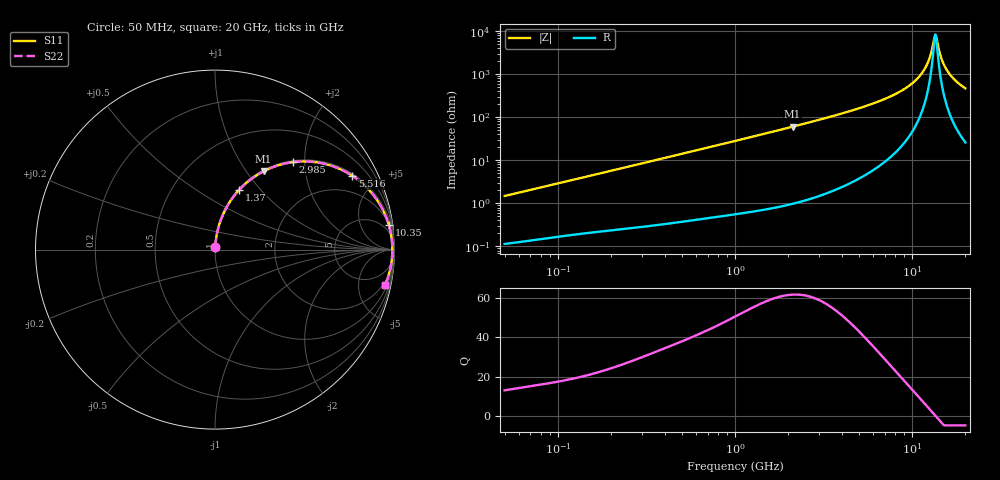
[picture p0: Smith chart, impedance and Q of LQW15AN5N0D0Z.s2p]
!Murata Part Number: LQW15AN5N0D0Z
!These Parameters are Measured in Series Mode Connection
!  o--[Z]--o
!Port1  Port2
!  o-------o
!Freq. Start=50[MHz] Stop=20[GHz], 401[Steps]
# Hz S RI R 50
!Freq.(Hz) S11(Real) S11(Imag) S21(Real) S21(Imag) S12(Real) S12(Imag) S22(Real) S22(Imag)
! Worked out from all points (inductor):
!   401 points, 50 MHz to 20 GHz, reference 50 ohm
!   read as one part in series: L = 4.68 nH near 51.52 MHz
!   highest Q = 61.9 at 2.115 GHz (marker M1), where L = 4.54 nH
!   self-resonance near 13.35 GHz
!   S11 on the Smith chart (normalised r, x): 50 MHz: 1.00, +0.03; 1.37 GHz: 1.01, +0.77; 2.985 GHz: 1.03, +1.75; 5.516 GHz: 1.09, +3.68; 10.35 GHz: 2, +14; 20 GHz: 1.52, -9.39
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5e7  0.00136 0.0147  0.9986 -0.0147  0.9986 -0.0147  0.00136 0.0147
1.364002e8  0.0035 0.0391  0.9965 -0.0391  0.9965 -0.0391  0.0035 0.0391
3.721004e8  0.014 0.1035  0.986 -0.1035  0.986 -0.1035  0.014 0.1035
1e9  0.0776 0.2579  0.9224 -0.2579  0.9224 -0.2579  0.0776 0.2579
1.369645e9  0.1341 0.3321  0.8659 -0.3321  0.8659 -0.3321  0.1341 0.3321
2.114743e9  0.2703 0.4361  0.7297 -0.4361  0.7297 -0.4361  0.2703 0.4361
2.728004e9  0.3869 0.4788  0.6131 -0.4788  0.6131 -0.4788  0.3869 0.4788
2.98453e9  0.4335 0.4872  0.5665 -0.4872  0.5665 -0.4872  0.4335 0.4872
5.515528e9  0.7659 0.4108  0.2341 -0.4108  0.2341 -0.4108  0.7659 0.4108
7.442007e9  0.8887 0.296  0.1113 -0.296  0.1113 -0.296  0.8887 0.296
8.907419e9  0.9396 0.2127  0.0604 -0.2127  0.0604 -0.2127  0.9396 0.2127
1.034674e10  0.9681 0.1385  0.0319 -0.1385  0.0319 -0.1385  0.9681 0.1385
1.131968e10  0.9793 0.0927  0.0207 -0.0927  0.0207 -0.0927  0.9793 0.0927
1.201863e10  0.9842 0.0619  0.0158 -0.0619  0.0158 -0.0619  0.9842 0.0619
1.257102e10  0.9866 0.0387  0.0134 -0.0387  0.0134 -0.0387  0.9866 0.0387
1.314879e10  0.988 0.0154  0.012 -0.0154  0.012 -0.0154  0.988 0.0154
1.354865e10  0.9882 -0.000136  0.0118 0.000136  0.0118 0.000136  0.9882 -0.000136
1.396067e10  0.988 -0.0157  0.012 0.0157  0.012 0.0157  0.988 -0.0157
1.482269e10  0.9861 -0.0467  0.0139 0.0467  0.0139 0.0467  0.9861 -0.0467
1.573793e10  0.9822 -0.0776  0.0178 0.0776  0.0178 0.0776  0.9822 -0.0776
1.747767e10  0.9706 -0.1313  0.0294 0.1313  0.0294 0.1313  0.9706 -0.1313
2e10  0.9468 -0.1986  0.0532 0.1986  0.0532 0.1986  0.9468 -0.1986
